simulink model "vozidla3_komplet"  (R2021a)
settings: Solver=VariableStepAuto  StartTime=0.0  StopTime=70  RelTol=1e-9
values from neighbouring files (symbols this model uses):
  A = A(1:(pocet_stavu),1:(pocet_stavu))    [appDekompLQR.m]    (also in appLQR.m = A(1:(2*N-1),1:(2*N-1)); appSYM.m = A(1:(2*N-1),1:(2*N-1)); appSZV.m = A(1:(2*N-1),1:(2*N-1)); central_LQR.m = A(1:(2*N-1),1:(2*N-1)))
  B = zeros(pocet_stavu,N)    [appDekompLQR.m]    (also in appLQR.m = zeros(2*N-1,N); appSYM.m = zeros(2*N-1,N); appSZV.m = zeros(2*N-1,N); central_LQR.m = zeros(2*N-1,N))
  C = eye(pocet_stavu)    [appDekompLQR.m]    (also in appLQR.m; appSYM.m; appSZV.m; central_LQR.m)
  conds0 = zeros(1,2*N-1)    [central_LQR.m]    (also in central_SYM.m; distri_STRUKTURAL.m = zeros(1,pocet_stavu); distri_SZV.m; porovnani_rizeni.m)
  D = zeros(pocet_stavu,N)    [appDekompLQR.m]    (also in appLQR.m; appSYM.m; appSZV.m; central_LQR.m)
  K = zeros(N,pocet_stavu)    [appDekompLQR.m]    (also in appSYM.m = [[0,-1/5,0,-3/20,0,-1/10,0,-1/20,0]; appSZV.m = [[-5/2,-3,7/4,1/2,0,0,0];[-1/7,-2/7,-7/2,-37/7,18/7,0,0];[0,; central_LQR.m = -K; central_SYM.m = [[0,-1/5,0,-3/20,0,-1/10,0,-1/20,0])

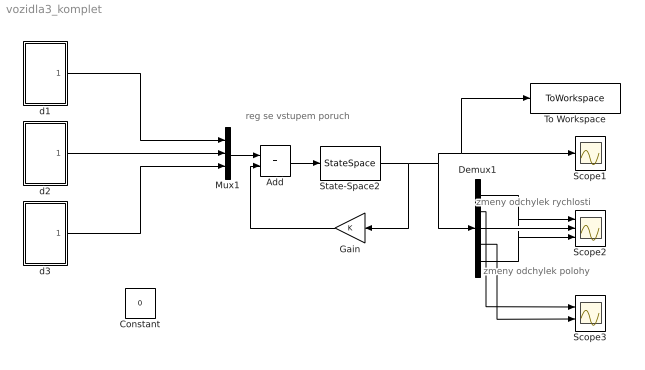
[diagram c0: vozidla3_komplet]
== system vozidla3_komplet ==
  note: zmeny odchylek rychlosti
  note: zmeny odchylek polohy
  note: reg se vstupem poruch
  Add : Sum
  Constant : Constant  Value=0
  Demux1 : Demux  Outputs=5
  Gain : Gain  Gain=K  Multiplication=Matrix(K*u)
  Mux1 : Mux  Inputs=3
  Scope1 : Scope
  Scope2 : Scope  NumInputPorts=3
  Scope3 : Scope  NumInputPorts=2
  State-Space2 : StateSpace  A=A  B=B  C=C  D=D  InitialCondition=conds0  ParameterTunability=Optimized
  To Workspace : ToWorkspace  VariableName=vystup  SaveFormat=Structure  SampleTime=-1
  d1 : Subsystem
  d2 : Subsystem
  d3 : Subsystem
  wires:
  Demux1/4 -> Scope3/2
  Demux1/3 -> Scope2/2
  Demux1/2 -> Scope3/1
  Demux1/5 -> Scope2/3
  Demux1/1 -> Scope2/1
  State-Space2/1 -> Gain/1, Demux1/1, Scope1/1, To Workspace/1
  Add/1 -> State-Space2/1
  Mux1/1 -> Add/1
  Gain/1 -> Add/2
  d1/1(Out1) -> Mux1/1
  d2/1(Out1) -> Mux1/2
  d3/1(Out1) -> Mux1/3

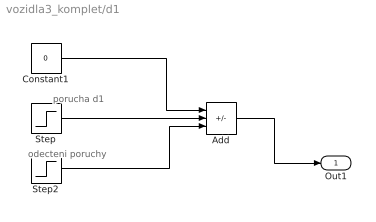
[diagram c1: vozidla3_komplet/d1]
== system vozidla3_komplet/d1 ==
  note: odecteni poruchy
  note: porucha d1
  Add : Sum  Inputs=++-
  Constant1 : Constant  Value=0
  Step : Step  Time=5  After=2  SampleTime=0
  Step2 : Step  Time=6  After=2  SampleTime=0
  Out1 : Outport
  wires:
  Constant1/1 -> Add/1
  Add/1 -> Out1/1
  Step/1 -> Add/2
  Step2/1 -> Add/3

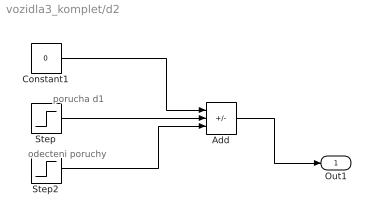
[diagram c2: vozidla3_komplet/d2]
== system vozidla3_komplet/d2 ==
  note: odecteni poruchy
  note: porucha d1
  Add : Sum  Inputs=++-
  Constant1 : Constant  Value=0
  Step : Step  Time=25  After=2  SampleTime=0
  Step2 : Step  Time=26  After=2  SampleTime=0
  Out1 : Outport
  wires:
  Constant1/1 -> Add/1
  Step2/1 -> Add/3
  Add/1 -> Out1/1
  Step/1 -> Add/2

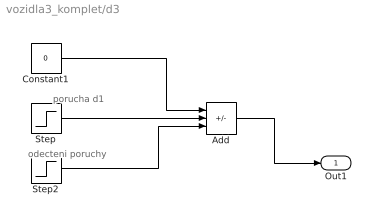
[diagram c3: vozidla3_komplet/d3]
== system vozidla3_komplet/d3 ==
  note: odecteni poruchy
  note: porucha d1
  Add : Sum  Inputs=++-
  Constant1 : Constant  Value=0
  Step : Step  Time=45  After=2  SampleTime=0
  Step2 : Step  Time=46  After=2  SampleTime=0
  Out1 : Outport
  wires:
  Constant1/1 -> Add/1
  Step2/1 -> Add/3
  Add/1 -> Out1/1
  Step/1 -> Add/2
